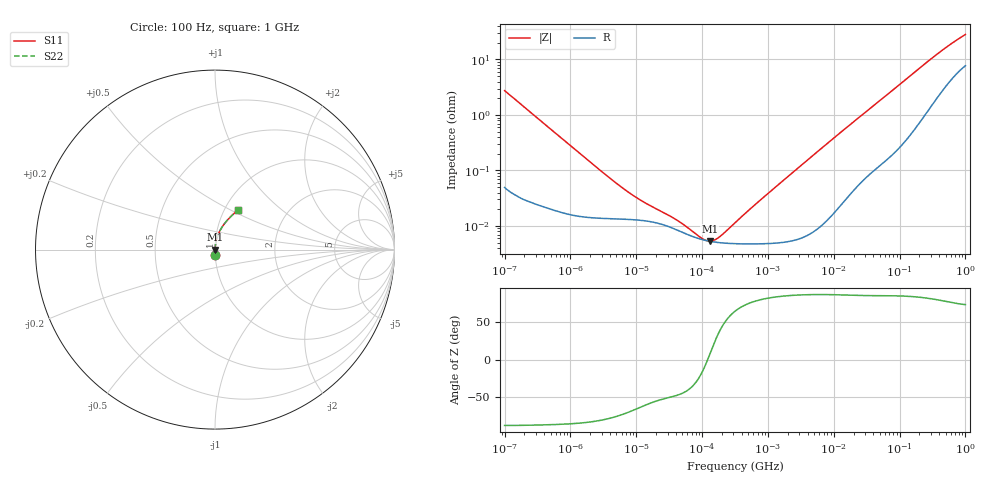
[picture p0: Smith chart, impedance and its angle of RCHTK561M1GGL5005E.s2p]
! RCHTK561M1GGL5005E  S-PARAMETER MODEL  (AEC-Q200 qualified)
! Model Generated by ELNA Corporation (http://www.ty-top.com)
! Version 1.0
! ELNA Control No. 240315
! Copyright (c) 2024 ELNA CO.,LTD. All Rights Reserved.
! Products Name : CONDUCTIVE POLYMER HYBRID ALUMINUM ELECTROLYTIC CAPACITORS
! Characteristics :
!  Capacitance  :  560uF  ,  Rated voltage  :  35V
!  Operating Temp. Range  :  -55 to +125 degC  ,  Endurance  :  4000hr at 125 degC
!  Dimension D  :  12.5mm  ,  Dimension L  :  13.5mm
! Frequency Range : 100Hz - 1GHz
! External Node Assignments :
!  1  o---| |---o  2
# MHz S RI R 50
!Freq[MHz].  S11 Real  S11 Imag  S21 Real  S21 Imag  S12 Real  S12 Imag  S22 Real  S22 Imag
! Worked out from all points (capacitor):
!   401 points, 100 Hz to 1 GHz, reference 50 ohm
!   read as one part in series: C = 578 uF near 108 Hz
!   lowest |Z| = 5.33 mohm at 130.3 kHz (marker M1)
!   series resonance near 121.7 kHz, so ESL is about 3 nH
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0.0001  0.00125 -0.0275  0.9988 0.0275  0.9988 0.0275  0.00125 -0.0275
0.000113  0.00103 -0.0244  0.999 0.0244  0.999 0.0244  0.00103 -0.0244
0.001488  0.00015 -0.00189  0.9999 0.00189  0.9999 0.00189  0.00015 -0.00189
0.003758  0.000136 -0.000754  0.9999 0.000754  0.9999 0.000754  0.000136 -0.000754
0.007161  0.000132 -0.000406  0.9999 0.000406  0.9999 0.000406  0.000132 -0.000406
0.012092  0.000126 -0.000254  0.9999 0.000254  0.9999 0.000254  0.000126 -0.000254
0.022131  0.000111 -0.000157  0.9999 0.000157  0.9999 0.000157  0.000111 -0.000157
0.034475  9.27e-05 -0.000112  0.9999 0.000112  0.9999 0.000112  9.27e-05 -0.000112
0.055911  7.26e-05 -6.86e-05  0.9999 6.86e-05  0.9999 6.86e-05  7.26e-05 -6.86e-05
0.060604  6.97e-05 -6.15e-05  0.9999 6.15e-05  0.9999 6.15e-05  6.97e-05 -6.15e-05
0.130317  5.29e-05 6.19e-06  0.9999 -6.19e-06  0.9999 -6.19e-06  5.29e-05 6.19e-06
0.258523  4.84e-05 7.7e-05  1 -7.7e-05  1 -7.7e-05  4.84e-05 7.7e-05
0.280221  4.82e-05 8.71e-05  1 -8.71e-05  1 -8.71e-05  4.82e-05 8.71e-05
0.316228  4.79e-05 0.000103  1 -0.000103  1 -0.000103  4.79e-05 0.000103
0.798914  4.77e-05 0.000301  1 -0.000301  1 -0.000301  4.77e-05 0.000301
4.704354  7.88e-05 0.00181  0.9999 -0.00181  0.9999 -0.00181  7.88e-05 0.00181
15.13561  0.00033 0.00574  0.9997 -0.00574  0.9997 -0.00574  0.00033 0.00574
69.9842  0.00232 0.0248  0.9977 -0.0248  0.9977 -0.0248  0.00232 0.0248
169.8244  0.00891 0.0582  0.9911 -0.0582  0.9911 -0.0582  0.00891 0.0582
365.1741  0.0329 0.115  0.9671 -0.115  0.9671 -0.115  0.0329 0.115
641.9482  0.0764 0.1723  0.9236 -0.1723  0.9236 -0.1723  0.0764 0.1723
1000  0.1271 0.2202  0.8729 -0.2202  0.8729 -0.2202  0.1271 0.2202
